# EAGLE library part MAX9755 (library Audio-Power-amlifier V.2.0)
The MAX9755 combine a stereo, 2.6W audio power amplifier and stereo DirectDrive® 110mW headphone amplifier in a single device. The headphone amplifier uses Maxim’s DirectDrive architecture that produces a ground-referenced output from a single supply, eliminating the need for large DC-blocking capacitors, saving cost, space, and component height. A high 90dB PSRR and low 0.01% THD+N ensures clean, low-distortion amplification of the audio signal.
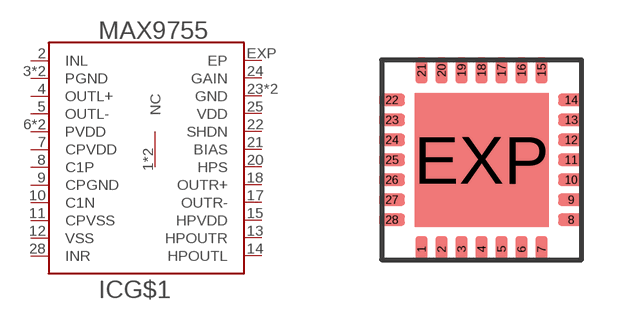
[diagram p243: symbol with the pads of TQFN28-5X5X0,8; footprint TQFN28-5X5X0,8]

Designator prefix IC; gates G$1=MAX9755 G$2=NC

## MAX9755  [TQFN28-5X5X0,8]
1  G$2:NC  nc
2  G$1:INL  in
3  G$1:PGND  pwr
4  G$1:OUTL+  out
5  G$1:OUTL-  out
6  G$1:PVDD  pwr
7  G$1:CPVDD  pwr
8  G$1:C1P
9  G$1:CPGND  pwr
10  G$1:C1N  in
11  G$1:CPVSS  pwr
12  G$1:VSS  pwr
13  G$1:HPOUTR  out
14  G$1:HPOUTL  out
15  G$1:HPVDD  pwr
16  G$1:PVDD  pwr
17  G$1:OUTR-  out
18  G$1:OUTR+  out
19  G$1:PGND  pwr
20  G$1:HPS  in
21  G$1:BIAS
22  G$1:SHDN
23  G$1:GND  pwr
24  G$1:GAIN  in
25  G$1:VDD  pwr
26  G$1:GND  pwr
27  G$2:NC  nc
28  G$1:INR  in
EXP  G$1:EP  pwr

## Footprint TQFN28-5X5X0,8 (pad centres in mm)
TQFN28-5x5x0,8 Source: www.maxim-ic.com/packages
smd 0.305 x 0.65: 1 -1.5,-2.24; 2 -1,-2.24; 3 -0.5,-2.24; 4 0,-2.24; 5 0.5,-2.24; 6 1,-2.24; 7 1.5,-2.24; 15 1.5,2.24; 16 1,2.24; 17 0.5,2.24; 18 0,2.24; 19 -0.5,2.24; 20 -1,2.24; 21 -1.5,2.24
smd 0.65 x 0.305: 8 2.24,-1.5; 9 2.24,-1; 10 2.24,-0.5; 11 2.24,0; 12 2.24,0.5; 13 2.24,1; 14 2.24,1.5; 22 -2.24,1.5; 23 -2.24,1; 24 -2.24,0.5; 25 -2.24,0; 26 -2.24,-0.5; 27 -2.24,-1; 28 -2.24,-1.5
smd 3.35 x 3.35: EXP 0,0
